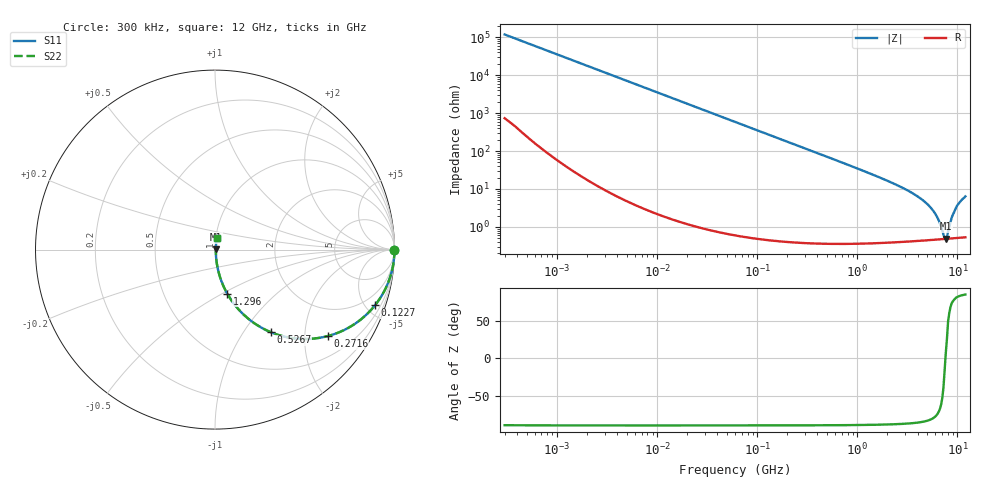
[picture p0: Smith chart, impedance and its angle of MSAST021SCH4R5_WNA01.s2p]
! MSAST021SCH4R5_WNA01  S-PARAMETER MODEL  ( General Type )
! Model Generated by TAIYO YUDEN Corporation (http://www.ty-top.com)
! Version 2.0
! TAIYO YUDEN Control No. 181101
! Copyright(c) 2015 TAIYO YUDEN CO.,LTD. All Rights Reserved.
! Product Description (link to TY-COMPAS)
! https://ds.yuden.co.jp/TYCOMPAS/or/detail?pn=MSAST021SCH4R5BWNA01&u=M
! Products Name : Multilayer Ceramic Capacitors
! Characteristics :
!  Capacitance : 4.5 pF , Rated Voltage : 25V , TCC : CH / C0H
!  Case Size : 0.25 x 0.125 / 0.0098 x 0.0049 [mm/inch] , Thickness : 0.125 / 0.0049 [mm/inch]
!  (Conditions: Temperature = 25 degC , DC Bias Current/Voltage = 0A / 0V)
! External Node Assignments :
!  1  o---| |---o  2
! GND o---------o GND
! Frequency Range : 0.3MHz  -  12000MHz  [ 401 STEP ]
# MHz S RI R 50
! Freq[MHz].  S11 Real  S11 Imag  S21 Real  S21 Imag  S12 Real  S12 Imag  S22 Real  S22 Imag
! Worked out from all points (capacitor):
!   401 points, 300 kHz to 12 GHz, reference 50 ohm
!   read as one part in series: C = 4.5 pF near 316.3 kHz
!   lowest |Z| = 489 mohm at 7.649 GHz (marker M1)
!   series resonance near 7.586 GHz, so ESL is about 98 pH
!   S11 on the Smith chart (normalised r, x): 300 kHz: open; 122.7 MHz: 1.01, -5.76; 271.6 MHz: 1.01, -2.60; 526.7 MHz: 1.01, -1.34; 1.296 GHz: 1.01, -0.53; 12 GHz: 1.01, +0.13
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0.3  1 -0.000848  6e-06 0.000848  6e-06 0.000848  1 -0.000848
1.769972  1 -0.005  3.03e-05 0.005  3.03e-05 0.005  1 -0.005
10.44266  0.9991 -0.0295  0.000889 0.0295  0.000889 0.0295  0.9991 -0.0295
60  0.9719 -0.1649  0.0281 0.1649  0.0281 0.1649  0.9719 -0.1649
122.6847  0.8922 -0.3094  0.1078 0.3094  0.1078 0.3094  0.8922 -0.3094
271.6094  0.6281 -0.4819  0.3719 0.4819  0.3719 0.4819  0.6281 -0.4819
353.9943  0.4985 -0.4982  0.5015 0.4982  0.5015 0.4982  0.4985 -0.4982
526.7124  0.3096 -0.4597  0.6904 0.4597  0.6904 0.4597  0.3096 -0.4597
804.7407  0.1609 -0.3633  0.8391 0.3633  0.8391 0.3633  0.1609 -0.3633
1296.429  0.0685 -0.2457  0.9315 0.2457  0.9315 0.2457  0.0685 -0.2457
2088.533  0.0275 -0.1515  0.9725 0.1515  0.9725 0.1515  0.0275 -0.1515
3547.679  0.0101 -0.0766  0.9899 0.0766  0.9899 0.0766  0.0101 -0.0766
5006.236  0.00598 -0.0392  0.994 0.0392  0.994 0.0392  0.00598 -0.0392
6026.253  0.00505 -0.0211  0.995 0.0211  0.995 0.0211  0.00505 -0.0211
6524.734  0.00486 -0.0136  0.9951 0.0136  0.9951 0.0136  0.00486 -0.0136
7254.098  0.00479 -0.00377  0.9952 0.00377  0.9952 0.00377  0.00479 -0.00377
7648.807  0.00482 0.000607  0.9952 -0.000607  0.9952 -0.000607  0.00482 0.000607
8064.993  0.00491 0.00572  0.9951 -0.00572  0.9951 -0.00572  0.00491 0.00572
8732.115  0.00522 0.0162  0.9948 -0.0162  0.9948 -0.0162  0.00522 0.0162
9454.42  0.00579 0.0274  0.9942 -0.0274  0.9942 -0.0274  0.00579 0.0274
10511.28  0.00708 0.0437  0.9929 -0.0437  0.9929 -0.0437  0.00708 0.0437
12000  0.00928 0.0627  0.9907 -0.0627  0.9907 -0.0627  0.00928 0.0627
